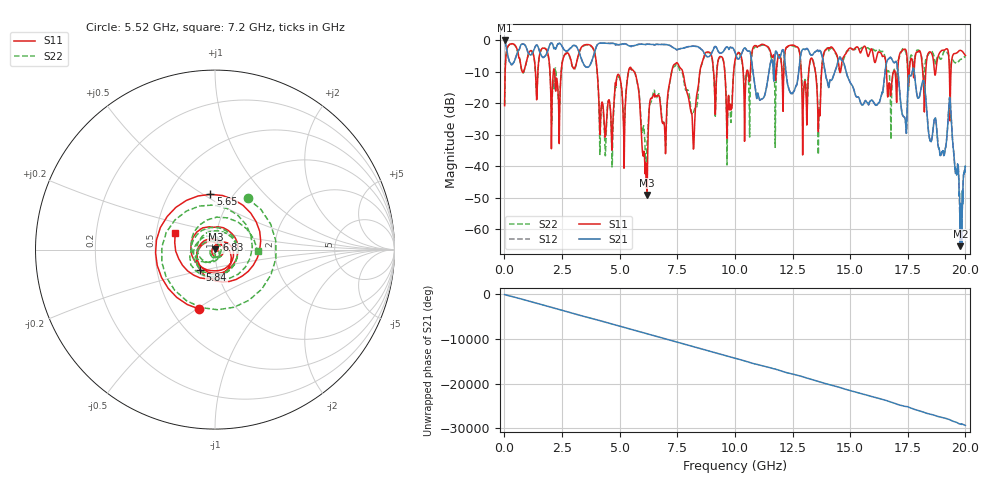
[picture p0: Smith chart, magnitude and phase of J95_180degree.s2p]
!Keysight Technologies,N5222A,MY51421036,A.10.65.16
!Date: Friday, March 31, 2023 14:18:00
!Correction: S11(Full 2 Port(1,2))
!S21(Full 2 Port(1,2))
!S12(Full 2 Port(1,2))
!S22(Full 2 Port(1,2))
!S2P File: Measurements: S11, S21, S12, S22:
# Hz S  dB  R 50
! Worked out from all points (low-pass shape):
!   2000 points, 10 MHz to 20 GHz, reference 50 ohm
!   highest |S21| = -0.14 dB at 10 MHz (marker M1); lowest = -65.3 dB at 19.78 GHz (marker M2)
!   |S21| within 3 dB of the highest: 1.895 GHz to 2.6 GHz (705.5 MHz wide, 31.4 % of centre); 3.945 GHz to 8.578 GHz (4.633 GHz wide, 74 % of centre)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
!   lowest |S11| = -49.1 dB at 6.19 GHz (marker M3), VSWR 1.01, Z = 50.3 + j0.234 ohm
!   |S11| at or under -10 dB: 4.026 GHz to 5.38 GHz (1.354 GHz wide, 28.8 % of centre); 5.632 GHz to 7.259 GHz (1.627 GHz wide, 25.2 % of centre); 7.734 GHz to 8.483 GHz (748.6 MHz wide, 9.23 % of centre)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
!   |S22| runs from -40.2 to -1.2 dB; largest |S21 - S12| = 0.0093
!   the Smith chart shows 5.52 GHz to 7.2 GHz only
!   S11 on the Smith chart (normalised r, x): 5.52 GHz: 0.68, -0.51; 5.65 GHz: 0.79, +0.54; 5.84 GHz: 0.83, -0.19; 6.83 GHz: 1.02, +0.11; 7.2 GHz: 0.63, +0.12
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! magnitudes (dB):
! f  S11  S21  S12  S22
! 10 MHz  -20.8  -0.1  -0.2  -20.7
! 3.35 GHz  -2.2  -6.2  -6.1  -2.4
! 4.37 GHz  -30.7  -1.0  -1.0  -35.5
! 5.52 GHz  -9.3  -1.9  -1.9  -9.4
! 5.65 GHz  -10.2  -1.8  -1.7  -10.1
! 5.84 GHz  -17.0  -1.4  -1.3  -16.4
! 6.19 GHz  -49.1  -1.3  -1.3  -33.7
! 6.68 GHz  -17.4  -1.4  -1.4  -17.1
! 6.83 GHz  -25.3  -1.4  -1.4  -24.6
! 7.2 GHz  -12.4  -1.8  -1.8  -12.5
! 8.18 GHz  -31.2  -1.9  -1.9  -23.4
! 8.73 GHz  -4.1  -4.9  -4.8  -4.3
! 9.74 GHz  -18.7  -3.0  -3.0  -17.8
! 10.01 GHz  -6.3  -3.9  -3.9  -6.7
! 11.15 GHz  -1.4  -18.8  -18.8  -1.7
! 13.34 GHz  -5.8  -4.8  -4.8  -5.8
! 15.53 GHz  -2.8  -20.6  -20.7  -2.4
! 16.67 GHz  -14.2  -6.0  -6.0  -9.8
! 18.97 GHz  -3.3  -35.5  -35.7  -5.8
! 19.33 GHz  -23.0  -18.3  -18.4  -10.2
! 19.78 GHz  -3.3  -65.3  -59.2  -6.2
! 20 GHz  -4.9  -40.0  -40.9  -5.6
